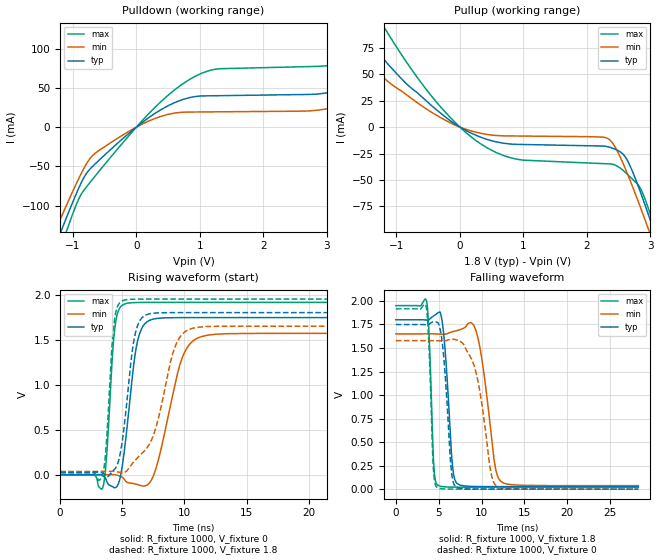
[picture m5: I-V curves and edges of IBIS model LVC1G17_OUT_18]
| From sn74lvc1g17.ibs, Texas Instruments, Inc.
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[Model]   LVC1G17_OUT_18
Model_type  Output
Vref =   0
Rref =   1000
Cref =   30p
Vmeas =   0.9
| variable   typ   min   max
C_comp   9.87pF   6.40pF   15.76pF
| C_pullup   9.16pF   6.40pF   10.36pF
| C_pulldown   10.57pF   6.59pF   15.76pF
[Temperature Range]   40   100   -40
| Ambient temperature   25   85   -40
[Voltage range]   1.8   1.65   1.95
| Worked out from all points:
|   slope of the pulldown table from 0 to 0.27 V, typ, clamps not added: 16.6 ohm
|   slope of the pullup table from 0 to 0.27 V, typ, clamps not added: 33 ohm
|   rising waveform, R_fixture 1000, V_fixture 0: 20-80 % time 867ps typ, 1.55ns min, 504ps max; typ from 0 V to 1.74 V
|   falling waveform, R_fixture 1000, V_fixture 1.8: 20-80 % time 717ps typ, 1.28ns min, 432ps max; typ from 1.8 V to 0.027 V
|   rising waveform, R_fixture 1000, V_fixture 1.8: 20-80 % time 874ps typ, 1.77ns min, 504ps max; typ from 0.027 V to 1.8 V
|   falling waveform, R_fixture 1000, V_fixture 0: 20-80 % time 749ps typ, 1.58ns min, 436ps max; typ from 1.75 V to 0 V
[Pulldown]
| LVC1G17_OUT_18
|   Voltage   I(typ)   I(min)   I(max)
-5.5V     -1.024A    -932.8mA   -1.143A
-1.25V    -145.7mA   -126.9mA   -167.2mA
-1.105V   -116mA     -100.2mA   -133.6mA
-650mV    -46.91mA   -33.3mA    -62.35mA
825mV     37.35mA    19.19mA    60.06mA
3.115V    45.49mA    25.17mA    79.66mA
3.755V    64.52mA    35.93mA    102.7mA
4.19V     79.14mA    21.53mA    128.2mA
4.47V     45.47mA    21.68mA    146.2mA
4.725V    44.49mA    21.83mA    131.7mA
5.01V     44.71mA    22mA       83.05mA
11V       50.72mA    25.33mA    92.94mA
[Pullup]
| LVC1G17_OUT_18
|   Voltage   I(typ)   I(min)   I(max)
-5.5V     449.7mA    254mA      638.5mA
-2.225V   143.3mA    107.6mA    207.3mA
-1.755V   105.1mA    78.04mA    153.5mA
-1.195V   63.95mA    46.44mA    94.81mA
-375mV    16.75mA    11.48mA    24.15mA
420mV     -11.47mA   -6.842mA   -19.31mA
2.34V     -18.76mA   -11.2mA    -34.79mA
2.645V    -32.43mA   -45.25mA   -45.19mA
2.84V     -61.19mA   -75.65mA   -57.82mA
2.99V     -86.8mA    -100.4mA   -81.09mA
3.08V     -102.8mA   -115.6mA   -97.77mA
11V       -1.709A    -1.61A     -1.847A
[Ramp]
| LVC1G17_OUT_18
| variable   typ   min   max
dV/dt_r   1.13/9.34E-10   1.02/1.66E-09   1.24/5.48E-10
dV/dt_f   1.11/7.65E-10   1.04/1.40E-09   1.20/4.56E-10
R_load = 1000
[Rising Waveform]
| LVC1G17_OUT_18
R_fixture =   1000
C_fixture =   0
L_fixture =   0
V_fixture =   0
V_fixture_min = 0
V_fixture_max = 0
|   Time   V(typ)   V(min)   V(max)
0s        112.7pV    7.663nV    3.037nV
3.43ns    -9.976mV   1.642mV    -141.3mV
3.72ns    -61.14mV   1.762mV    178.1mV
4.38ns    -144mV     242.8uV    1.605V
5.105ns   200.8mV    -40.14mV   1.89V
6.14ns    1.424V     -105.6mV   1.912V
7.165ns   1.712V     -94.43mV   1.913V
9.7ns     1.744V     1.25V      1.913V
10.93ns   1.744V     1.508V     1.913V
28.3ns    1.744V     1.569V     1.913V
[Falling Waveform]
| LVC1G17_OUT_18
R_fixture =   1000
C_fixture =   0
L_fixture =   0
V_fixture =   1.8
V_fixture_min = 1.65
V_fixture_max = 1.95
|   Time   V(typ)   V(min)   V(max)
0s        1.8V       1.65V      1.95V
3.59ns    1.797V     1.65V      1.995V
4.42ns    1.841V     1.65V      267.9mV
4.885ns   1.873V     1.648V     43.12mV
5.515ns   1.707V     1.646V     26.51mV
6.585ns   274.6mV    1.672V     21.85mV
7.17ns    58.71mV    1.686V     21.38mV
9.42ns    28.41mV    1.664V     21.1mV
12.29ns   27.07mV    80.62mV    21.09mV
28.3ns    26.98mV    37.16mV    21.09mV
[Rising Waveform]
| LVC1G17_OUT_18
R_fixture =   1000
C_fixture =   0
L_fixture =   0
V_fixture =   1.8
V_fixture_min = 1.65
V_fixture_max = 1.95
|   Time   V(typ)   V(min)   V(max)
0s        26.95mV    37.1mV     21.07mV
3.375ns   21.98mV    38.58mV    -24.31mV
3.69ns    -6.583mV   38.61mV    299.8mV
4.32ns    52.68mV    37.61mV    1.662V
4.99ns    364.6mV    24.06mV    1.929V
5.96ns    1.51V      148.7mV    1.949V
6.905ns   1.774V     283.6mV    1.95V
9.19ns    1.8V       1.399V     1.95V
10.32ns   1.8V       1.61V      1.95V
28.3ns    1.8V       1.65V      1.95V
[Falling Waveform]
| LVC1G17_OUT_18
R_fixture =   1000
C_fixture =   0
L_fixture =   0
V_fixture =   0
V_fixture_min = 0
V_fixture_max = 0
|   Time   V(typ)   V(min)   V(max)
0s        1.749V     1.578V     1.916V
3.55ns    1.747V     1.578V     1.937V
4.375ns   1.778V     1.578V     232.8mV
4.805ns   1.774V     1.577V     19.23mV
5.435ns   1.543V     1.576V     4.304mV
6.445ns   229.2mV    1.593V     608uV
7ns       25.11mV    1.588V     242.3uV
9.265ns   710.3uV    1.272V     26.21uV
11.74ns   80.33uV    32.49mV    19.51uV
28.3ns    21.84uV    43.84uV    13.47uV
